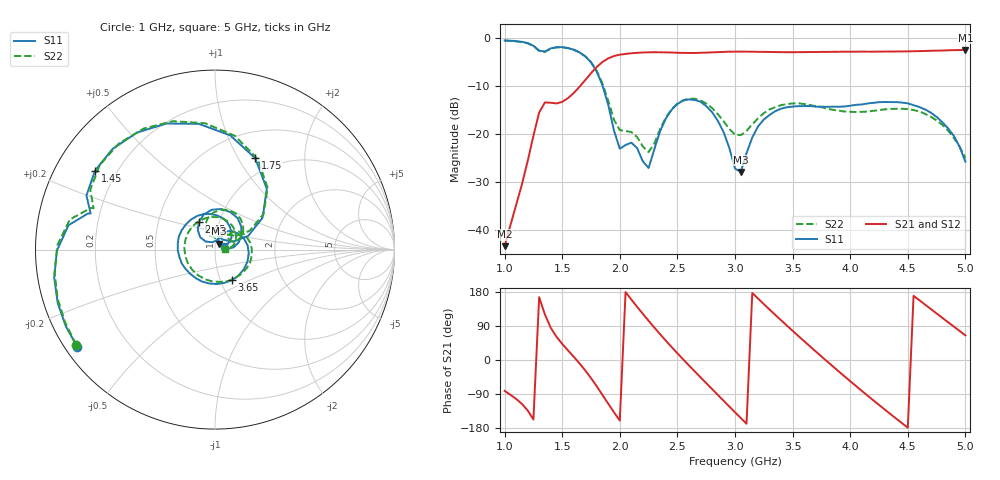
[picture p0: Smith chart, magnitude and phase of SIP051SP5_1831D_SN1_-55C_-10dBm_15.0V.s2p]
# GHz  S  dB  R  50
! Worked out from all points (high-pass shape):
!   81 points, 1 GHz to 5 GHz, reference 50 ohm
!   highest |S21| = -2.51 dB at 5 GHz (marker M1); lowest = -43.4 dB at 1 GHz (marker M2)
!   |S21| within 3 dB of the highest: 1.826 GHz to end of sweep
!   lowest |S11| = -27.9 dB at 3.05 GHz (marker M3), VSWR 1.08, Z = 52.1 + j3.52 ohm
!   |S11| at or under -10 dB: 1.851 GHz to end of sweep
!   |S22| runs from -25.0 to -0.6 dB; largest |S21 - S12| = 0.0018
!   S11 on the Smith chart (normalised r, x): 1 GHz: 0.03, -0.32; 1.45 GHz: 0.12, +0.30; 1.75 GHz: 0.80, +1.18; 2.45 GHz: 0.80, +0.25; 3.65 GHz: 1.14, -0.40; 5 GHz: 1.10, +0.04
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1  -0.54 -144.9  -43.38 -81.5  -43.23 -83.8  -0.56 -145.7
1.3  -2.67 164.1  -15.55 165.9  -15.54 166.0  -2.73 161.5
1.45  -1.94 146.7  -13.65 61.4  -13.65 61.4  -1.98 143.7
1.7  -3.85 82.4  -8.79 -27.5  -8.79 -27.4  -3.83 80.1
1.75  -5.09 66.3  -7.35 -47.8  -7.36 -47.7  -5.06 64.8
1.9  -13.99 22.3  -4.26 -115.6  -4.26 -115.5  -13.10 28.5
2.05  -22.32 74.6  -3.35 179.4  -3.34 179.4  -19.39 59.8
2.25  -27.09 113.2  -3.01 103.5  -3.00 103.5  -23.77 87.6
2.35  -19.42 140.3  -3.00 68.0  -2.98 68.0  -18.96 115.0
2.45  -14.97 120.4  -3.05 34.1  -3.06 34.1  -14.85 102.8
2.6  -12.81 81.4  -3.15 -14.3  -3.13 -14.3  -12.67 71.5
2.75  -14.19 41.6  -3.07 -61.0  -3.07 -60.9  -13.66 41.0
3  -27.21 17.1  -2.87 -137.9  -2.87 -137.9  -20.15 30.2
3.05  -27.93 57.1  -2.87 -153.1  -2.85 -153.1  -20.26 39.6
3.2  -18.45 58.3  -2.91 162.1  -2.90 162.1  -16.76 43.7
3.4  -14.74 7.3  -2.97 104.9  -2.96 104.8  -14.01 11.5
3.65  -14.20 -60.7  -2.94 36.2  -2.95 36.3  -13.97 -41.6
3.7  -14.31 -74.0  -2.95 22.8  -2.94 22.8  -14.22 -54.4
4.05  -13.94 -157.7  -2.88 -68.6  -2.87 -68.7  -15.43 -153.1
4.35  -13.38 139.1  -2.85 -142.9  -2.86 -142.8  -14.81 121.8
4.65  -14.91 75.6  -2.73 146.2  -2.73 146.1  -15.82 51.8
5  -25.77 22.4  -2.51 65.0  -2.51 64.9  -24.98 5.4
